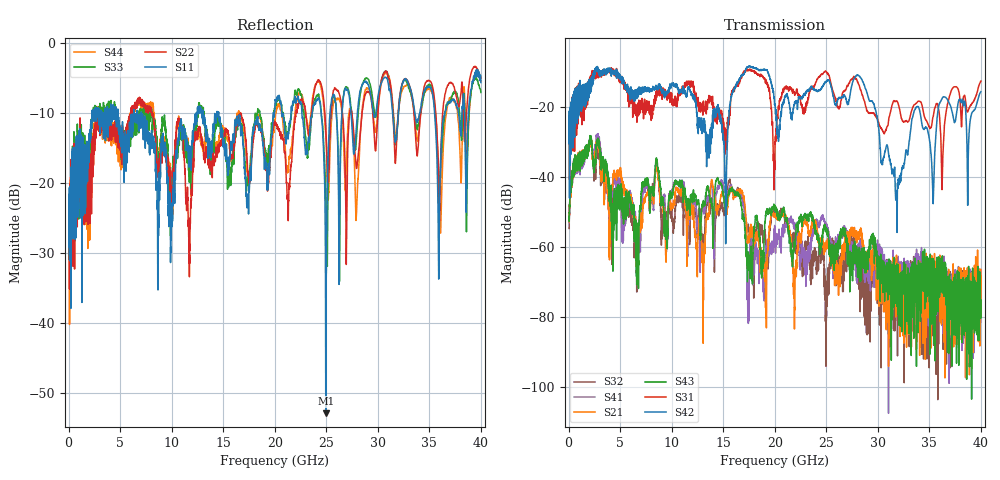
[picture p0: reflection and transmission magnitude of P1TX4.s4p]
!Agilent Technologies,N5245A,MY49151084,A.09.20.08
!Agilent N5245A: A.09.20.08
!Date: Thursday, March 01, 2012 14:37:39
!Correction: S11(Full 4 Port(1,2,3,4))
!S12(Full 4 Port(1,2,3,4))
!S13(Full 4 Port(1,2,3,4))
!S14(Full 4 Port(1,2,3,4))
!S21(Full 4 Port(1,2,3,4))
!S22(Full 4 Port(1,2,3,4))
!S23(Full 4 Port(1,2,3,4))
!S24(Full 4 Port(1,2,3,4))
!S31(Full 4 Port(1,2,3,4))
!S32(Full 4 Port(1,2,3,4))
!S33(Full 4 Port(1,2,3,4))
!S34(Full 4 Port(1,2,3,4))
!S41(Full 4 Port(1,2,3,4))
!S42(Full 4 Port(1,2,3,4))
!S43(Full 4 Port(1,2,3,4))
!S44(Full 4 Port(1,2,3,4))
!S4P File: Measurements: <S11,S12,S13,S14>,
!<S21,S22,S23,S24>,
!<S31,S32,S33,S34>,
!<S41,S42,S43,S44>:
# Hz S  dB  R 50
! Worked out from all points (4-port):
!   3996 points, 50 MHz to 40 GHz, reference 50 ohm
!   strongest paths, dB at 50 MHz, 10.04 GHz, 20.03 GHz, 30.02 GHz, 40 GHz:
!     S42: -25.3, -13.4, -19.3, -24.8, -15.7
!     S31: -26.4, -18.5, -30.0, -23.9, -12.7
!     S43: -51.3, -45.2, -48.6, -69.1, -75.1
!     S21: -52.6, -48.5, -51.2, -73.3, -66.4
!     S41: -52.6, -43.9, -56.3, -59.5, -81.5
!     S32: -54.7, -50.8, -50.4, -66.4, -75.4
!   lowest |S11| = -52.9 dB at 24.95 GHz (marker M1), VSWR 1.00, Z = 49.8 + j0.0115 ohm
!   |S11| at or under -10 dB: start of sweep to 2.256 GHz; 7.051 GHz to 12.46 GHz (5.406 GHz wide, 55.4 % of centre); 14.56 GHz to 19.86 GHz (5.295 GHz wide, 30.8 % of centre)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
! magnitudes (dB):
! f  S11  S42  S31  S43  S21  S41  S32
! 50 MHz  -24.6  -25.3  -26.4  -51.3  -52.6  -52.6  -54.7
! 15.63 GHz  -16.7  -19.5  -22.2  -43.7  -44.4  -43.1  -40.9
! 17.43 GHz  -21.6  -8.5  -9.3  -63.2  -57.5  -76.9  -53.9
! 19.99 GHz  -9.7  -19.2  -37.6  -48.5  -51.0  -53.8  -51.3
! 24.95 GHz  -52.9  -12.9  -9.8  -54.7  -59.4  -53.9  -81.5
! 31.87 GHz  -12.2  -55.8  -18.4  -72.4  -69.2  -70.3  -79.8
! 40 GHz  -5.6  -15.7  -12.7  -75.1  -66.4  -81.5  -75.4
